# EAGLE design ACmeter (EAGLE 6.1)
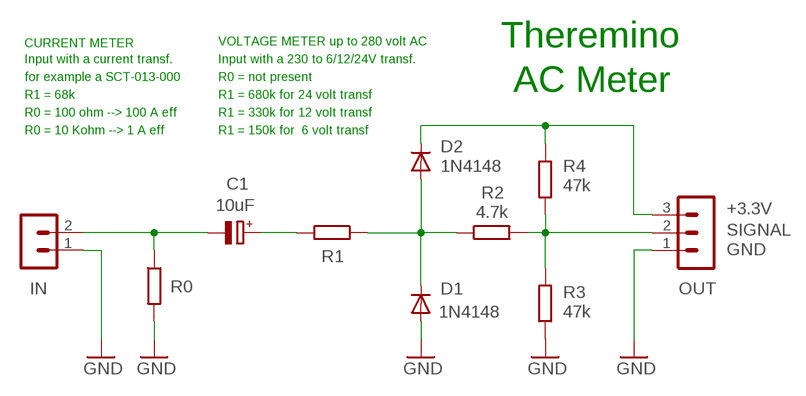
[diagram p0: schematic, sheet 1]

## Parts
C1  10uF  CPOL-EUE2-5B  [E2-5B]
D1  1N4148  DIODE-DO34-7  [DO34-7]
D2  1N4148  DIODE-DO34-7  [DO34-7]
IN  MA02-1N  [MA02-1]
OUT  MA03-1L3  [MA03-1_L3]
R0  See text  R-EU_0204/7  [0204/7]
R1  see text  R-EU_0204/7  [0204/7]
R2  4.7k  R-EU_0204/7  [0204/7]
R3  47k  R-EU_0204/7  [0204/7]
R4  47k  R-EU_0204/7  [0204/7]

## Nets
GND: D1.A IN.1 OUT.1 R0.2 R3.1
N$2: D1.C D2.A R1.1 R2.1
N$3: OUT.2 R2.2 R3.2 R4.2
N$4: D2.C OUT.3 R4.1
N$5: C1.- IN.2 R0.1
N$6: C1.+ R1.2

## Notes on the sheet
- CURRENT METER | VOLTAGE METER up to 280 volt AC | Theremino
- Input with a current transf. | Input with a 230 to 6/12/24V transf.
- for example a SCT-013-000 | R0 = not present
- AC Meter
- R1 = 68k | R1 = 680k for 24 volt transf
- R0 = 100 ohm --> 100 A eff | R1 = 330k for 12 volt transf
- R0 = 10 Kohm --> 1 A eff | R1 = 150k for  6 volt transf
- +3.3V
- SIGNAL
- GND

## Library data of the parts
C1 = 00-LIVIO:CPOL-EU: POLARIZED CAPACITOR, European symbol
D1 D2 = 00-LIVIO:DIODE-: DIODE
IN = 03-con-lstb-M:MA02-1: PIN HEADER
OUT = 03-con-lstb-M:MA03-1: PIN HEADER
R0 R1-R4 = 00-LIVIO:R-EU_: RESISTOR, European symbol

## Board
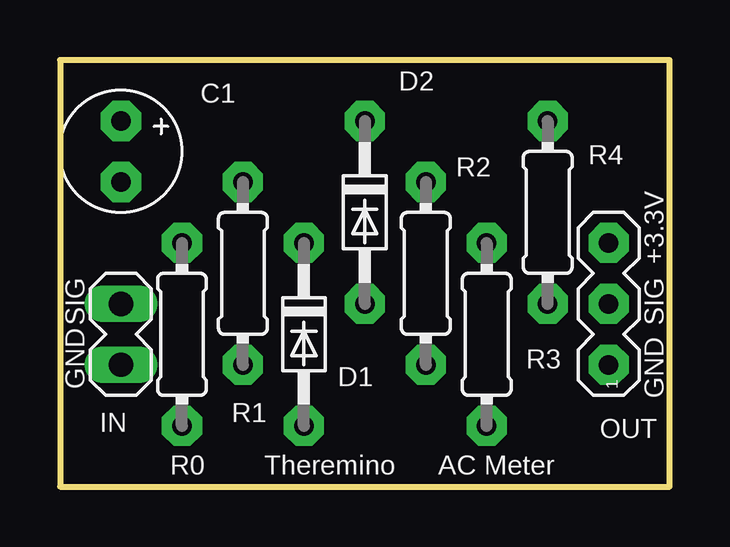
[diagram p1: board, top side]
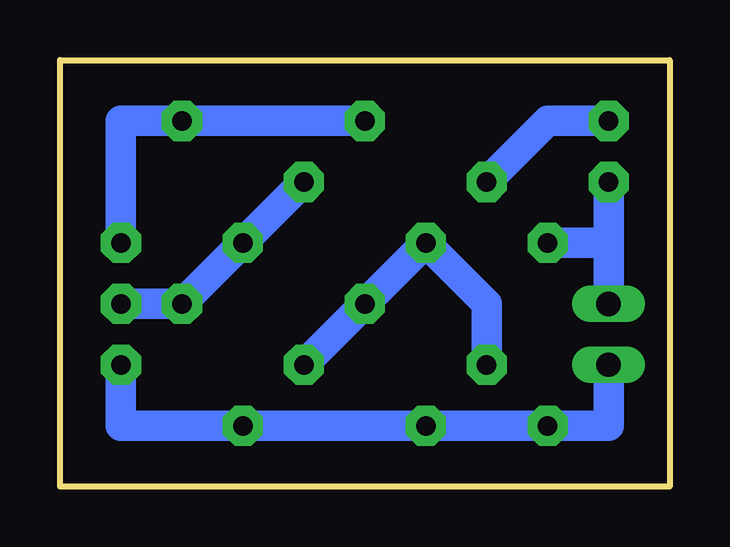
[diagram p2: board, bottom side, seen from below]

Size 25.4 x 17.78 mm. Coordinates in mm from the lower left corner, seen from the top.
Outline: 0,0 25.4,0 25.4,17.78 0,17.78 0,0
Copper layers (1*16): Top 0.035mm / dielectric 1.5mm / Bottom 0.035mm
Design rules: minimum track width 10mil, minimum drill 31mil, track to track 31mil, track to pad 31mil, pad to pad 31mil, via to via 31mil, smd to smd 31mil, copper to edge 31mil, drill to drill 8mil, minimum pad ring 5mil, minimum via ring 8mil, stop-mask expansion 4mil, vias tented up to drill 0mil, thermal gap 47mil

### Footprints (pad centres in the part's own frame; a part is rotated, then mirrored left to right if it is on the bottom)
E2-5B = drill 0.813 pad 1.676 octagon: + -1.27,0; - 1.27,0
DO34-7 = drill 0.813 pad 1.676 octagon: A 3.81,0; C -3.81,0
MA02-1 = drill 1.016 long: 1 -1.27,0; 2 1.27,0
MA03-1_L3 = drill 0.813 pad 1.676 octagon: 1 -2.54,0; 2 0,0; 3 2.54,0
0204/7 = drill 0.813 pad 1.676 octagon: 1 -3.81,0; 2 3.81,0

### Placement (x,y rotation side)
C1  2.54,13.97 270 top
D1  10.16,6.35 270 top
D2  12.7,11.43 270 top
IN  2.54,6.35 90 top
OUT  22.86,7.62 90 top
R0  5.08,6.35 270 top
R1  7.62,8.89 90 top
R2  15.24,8.89 90 top
R3  17.78,6.35 90 top
R4  20.32,11.43 270 top

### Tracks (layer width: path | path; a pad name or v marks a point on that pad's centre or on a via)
GND
  Bottom 1.27: OUT.1 22.86,2.54 R3.1 D1.A R0.2 2.54,2.54 IN.1
N$1
  Bottom 1.27: 2.54,15.24 5.08,15.24
N$2
  Bottom 1.27: R2.1 D2.A D1.C 7.62,7.62 R1.1
N$3
  Bottom 1.27: OUT.2 R4.2 R3.2 R2.2
N$4
  Bottom 1.27: D2.C R4.1 22.86,15.24 OUT.3
N$5
  Bottom 1.27: C1.- IN.2 2.54,10.16 R0.1
N$6
  Bottom 1.27: C1.+ 5.08,15.24 R1.2

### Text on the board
tNames: +3.3V | SIG | SIG | GND | GND | Theremino | AC Meter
